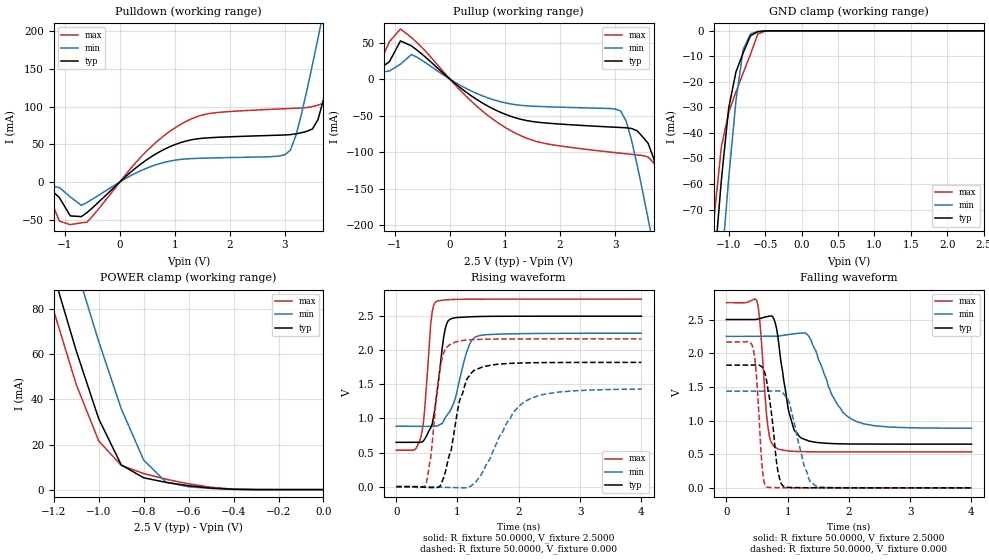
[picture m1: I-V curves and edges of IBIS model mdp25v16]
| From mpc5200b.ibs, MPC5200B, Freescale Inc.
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|   Model mdp25v16
[Model]   mdp25v16
Model_type   I/O
Polarity   Non-Inverting
Enable   Active-High
Vinl =   0.8000V
Vinh =   2.0000V
Vmeas =   1.5000V
C_comp   2.1096pF   1.4802pF   2.7108pF
[Temperature Range]   27.0000   0.1250k   -40.0000
[Voltage Range]   2.5000V   2.2500V   2.7500V
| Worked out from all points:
|   slope of the pulldown table from 0 to 0.375 V, typ, clamps not added: 16 ohm
|   slope of the pullup table from 0 to 0.375 V, typ, clamps not added: 17 ohm
|   GND clamp passes 1 mA (typ) near -0.64 V on its own axis
|   POWER clamp passes 1 mA (typ) near -0.53 V on its own axis
|   rising waveform, R_fixture 50.0000, V_fixture 2.5000: 20-80 % time 157ps typ, 248ps min, 108ps max; typ from 0.649 V to 2.5 V
|   rising waveform, R_fixture 50.0000, V_fixture 0.000: 20-80 % time 272ps typ, 518ps min, 155ps max; typ from 0 V to 1.82 V
|   falling waveform, R_fixture 50.0000, V_fixture 2.5000: 20-80 % time 199ps typ, 397ps min, 108ps max; typ from 2.5 V to 0.649 V
|   falling waveform, R_fixture 50.0000, V_fixture 0.000: 20-80 % time 142ps typ, 226ps min, 89.3ps max; typ from 1.82 V to 0 V
[Pulldown]
| voltage   I(typ)   I(min)   I(max)
-2.5V     -2.01mA    -1.636mA   -1.932mA
-1.5V     -4.426mA   -3.227mA   -6.191mA
-1.1V     -20.76mA   -7.457mA   -51.97mA
-600mV    -40.91mA   -27.44mA   -53.5mA
1.1V      52.15mA    29.86mA    76.28mA
3V        62.36mA    36.04mA    97.26mA
3.2V      63.89mA    61.99mA    97.91mA
3.5V      70.36mA    156mA      100.1mA
3.7V      109.5mA    226.3mA    104.4mA
4V        211.9mA    335mA      124mA
4.4V      360.1mA    482.7mA    256.5mA
5V        589.8mA    707.5mA    487.1mA
[Pullup]
| voltage   I(typ)   I(min)   I(max)
-2.5V     5.715mA    6.879mA    5.147mA
-1.3V     13.27mA    8.942mA    18.03mA
-900mV    52.46mA    20.58mA    68.85mA
-700mV    45.64mA    33.81mA    57.05mA
1.1V      -50.75mA   -33.86mA   -70.42mA
3.1V      -66.17mA   -43.61mA   -101.4mA
3.3V      -67.6mA    -84.01mA   -103mA
3.6V      -87.85mA   -191.3mA   -106.5mA
3.7V      -108.4mA   -230mA     -114.8mA
4V        -214.4mA   -348.9mA   -139mA
4.4V      -373.4mA   -510.8mA   -253.6mA
5V        -618.9mA   -756.9mA   -495.9mA
[GND_clamp]
| voltage   I(typ)   I(min)   I(max)
-2.5V     -616.3mA   -652.4mA   -595.9mA
-1.3V     -130.6mA   -168mA     -108.6mA
-1.2V     -93.21mA   -129.8mA   -73.24mA
-1.1V     -58.45mA   -92.8mA    -45.46mA
-1V       -30.33mA   -57.91mA   -32.05mA
-900mV    -16.1mA    -27.42mA   -23.9mA
-800mV    -8.518mA   -7.241mA   -16.44mA
-700mV    -1.909mA   -1.177mA   -9.176mA
-600mV    -364.7uA   -212.2uA   -1.283mA
-500mV    -39.19uA   -34.54uA   -92.63uA
2.5V      257.5pA    5.084uA    26.52pA
[POWER_clamp]
| voltage   I(typ)   I(min)   I(max)
-2.5V     584.4mA    609.4mA    577.7mA
-1.3V     130.2mA    167.4mA    114.6mA
-1.2V     95.06mA    132.3mA    79.13mA
-1.1V     61.46mA    98.2mA     46.53mA
-1V       31.32mA    65.57mA    21.52mA
-900mV    10.96mA    35.88mA    10.75mA
-800mV    5.231mA    13.06mA    7.129mA
-700mV    3.197mA    3.28mA     4.595mA
-600mV    1.712mA    1.263mA    2.547mA
-500mV    672.1uA    514.1uA    1.035mA
-400mV    127.3uA    134.7uA    183.8uA
0V        257.5pA    3.062nA    43.96pA
[Ramp]
| variable   typ   min   max
dV/dt_r   1.0910/0.2550n   0.7965/0.4516n   1.2997/0.1531n
dV/dt_f   1.1100/0.1951n   0.7854/0.3656n   1.3295/0.1073n
R_load = 50.0000
[Rising Waveform]
R_fixture = 50.0000
V_fixture = 2.5000
V_fixture_min = 2.2500
V_fixture_max = 2.7500
| time   V(typ)   V(min)   V(max)
0s        649.3mV    885.4mV    534.1mV
399ps     650.4mV    885.7mV    713.1mV
469.4ps   702.9mV    885.7mV    1.187V
563.3ps   862mV      884.1mV    2.395V
657.1ps   1.326V     887mV      2.717V
774.5ps   2.195V     967.2mV    2.736V
891.8ps   2.46V      1.131V     2.743V
1.15ns    2.489V     1.971V     2.748V
1.291ns   2.494V     2.195V     2.749V
4ns       2.5V       2.25V      2.75V
[Rising Waveform]
R_fixture = 50.0000
V_fixture = 0.000
| time   V(typ)   V(min)   V(max)
0s        8.205nV    105.3nV    11.71nV
492.9ps   -13.43mV   385uV      57.83mV
563.3ps   -13.49mV   303.3uV    427.2mV
727.6ps   26.62mV    -5.326mV   1.783V
891.8ps   506.7mV    -11mV      2.094V
1.033ns   1.256V     -16.07mV   2.135V
1.267ns   1.702V     43.81mV    2.157V
1.901ns   1.809V     1.081V     2.166V
2.112ns   1.816V     1.254V     2.166V
4ns       1.822V     1.431V     2.166V
[Falling Waveform]
R_fixture = 50.0000
V_fixture = 2.5000
V_fixture_min = 2.2500
V_fixture_max = 2.7500
| time   V(typ)   V(min)   V(max)
0s        2.5V       2.25V      2.75V
492.9ps   2.503V     2.25V      2.792V
539.8ps   2.511V     2.25V      2.536V
680.6ps   2.546V     2.249V     893.4mV
798ps     2.45V      2.25V      600.2mV
1.009ns   1.17V      2.276V     548.7mV
1.22ns    741mV      2.298V     537.5mV
1.361ns   692.5mV    2.227V     535.5mV
2.042ns   651.3mV    1.022V     534.2mV
4ns       649.3mV    885.8mV    534.1mV
[Falling Waveform]
R_fixture = 50.0000
V_fixture = 0.000
| time   V(typ)   V(min)   V(max)
0s        1.822V     1.435V     2.166V
422.4ps   1.823V     1.435V     2.115V
492.9ps   1.827V     1.435V     1.643V
586.7ps   1.793V     1.435V     283.3mV
657.1ps   1.591V     1.436V     14.06mV
844.9ps   227.9mV    1.441V     2.661mV
938.8ps   20.65mV    1.395V     1.469mV
1.267ns   2.161mV    334.2mV    201uV
1.455ns   992.1uV    30.01mV    56.43uV
4ns       1.975uV    6.433uV    -1.955uV
